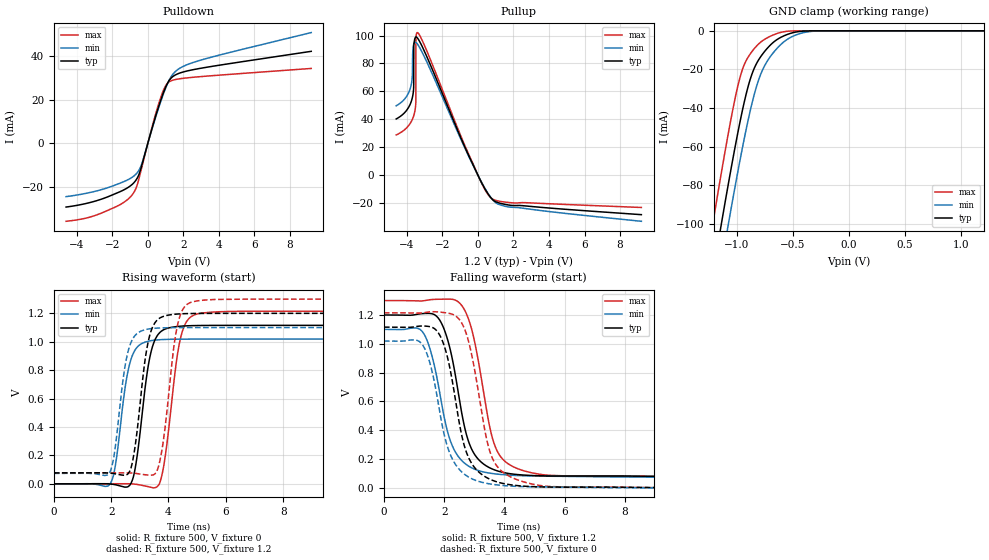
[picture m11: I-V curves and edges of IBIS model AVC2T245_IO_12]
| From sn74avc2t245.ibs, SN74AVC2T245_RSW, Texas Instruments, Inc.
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[Model]   AVC2T245_IO_12
Model_type  I/O
Vinl=0.385
Vinh=0.845
Enable   Active-Low
Vref =   0
Rref =   2000
Cref =   15p
Vmeas =   0.6
| variable   typ   min   max
C_comp   5.09pF   4.44pF   5.69pF
| C_pullup   5.41pF   3.52pF   7.45pF
| C_pulldown   4.96pF   4.40pF   6.21pF
| C_tri-state   5.09pF   4.44pF   5.69pF
[Temperature Range]   40   100   -40
| Ambient temperature   25   85   -40
[Voltage range]   1.2   1.1   1.3
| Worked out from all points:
|   slope of the pulldown table from 0 to 0.18 V, typ, clamps not added: 34.6 ohm
|   slope of the pullup table from 0 to 0.18 V, typ, clamps not added: 38.5 ohm
|   GND clamp passes 1 mA (typ) near -0.50 V on its own axis
|   rising waveform, R_fixture 500, V_fixture 0: 20-80 % time 426ps typ, 410ps min, 445ps max; typ from 0 V to 1.12 V
|   falling waveform, R_fixture 500, V_fixture 1.2: 20-80 % time 663ps typ, 677ps min, 669ps max; typ from 1.2 V to 0.077 V
|   rising waveform, R_fixture 500, V_fixture 1.2: 20-80 % time 407ps typ, 391ps min, 423ps max; typ from 0.077 V to 1.2 V
|   falling waveform, R_fixture 500, V_fixture 0: 20-80 % time 659ps typ, 674ps min, 671ps max; typ from 1.12 V to 0 V
[GND Clamp]
| AVC2T245_IO_12
|   Voltage   I(typ)   I(min)   I(max)
-4.6V     -1.415A    -1.424A    -1.406A
-1.23V    -132.8mA   -153.7mA   -106.4mA
-1.205V   -124mA     -145mA     -97.63mA
-1.135V   -99.98mA   -121mA     -73.45mA
-1.08V    -81.59mA   -102.5mA   -55.25mA
-1.065V   -76.69mA   -97.53mA   -50.48mA
-960mV    -44.57mA   -64.28mA   -22.28mA
-855mV    -21.19mA   -35.79mA   -10.15mA
-740mV    -9.962mA   -17.01mA   -4.06mA
-565mV    -2.263mA   -5.08mA    -343.5uA
-280mV    -5.263uA   -97.56uA   -11.86nA
1.2V      717.1pA    866.1nA    57.51pA
[Pulldown]
| AVC2T245_IO_12
|   Voltage   I(typ)   I(min)   I(max)
-4.6V     -28.98mA   -24.24mA   -35.47mA
-2.64V    -25.46mA   -21.11mA   -31.83mA
-1.485V   -21.69mA   -17.85mA   -27.52mA
-865mV    -18.55mA   -15.32mA   -23.28mA
-620mV    -16.14mA   -13.56mA   -19.46mA
-375mV    -11.06mA   -10.1mA    -12.1mA
650mV     17.79mA    17.17mA    19mA
955mV     24.67mA    24.15mA    25.54mA
1.215V    28.82mA    29mA       28.13mA
1.685V    31.71mA    33.63mA    29.31mA
2.565V    33.61mA    36.91mA    30.15mA
9.2V      41.96mA    50.5mA     34.16mA
[Pullup]
| AVC2T245_IO_12
|   Voltage   I(typ)   I(min)   I(max)
-4.6V     40.27mA    49.7mA     28.8mA
-3.925V   48.11mA    58.42mA    35.16mA
-3.69V    55.6mA     72.23mA    40.01mA
-3.67V    56.81mA    87.93mA    40.6mA
-3.615V   63.37mA    93.79mA    42.54mA
-3.61V    92.97mA    93.99mA    42.74mA
-3.555V   97.57mA    95.14mA    45.5mA
-3.495V   98.98mA    95.13mA    52.19mA
-3.49V    99mA       95.09mA    98.25mA
-3.4V     98.18mA    93.83mA    102.1mA
760mV     -16.62mA   -16.55mA   -16.53mA
9.2V      -28.27mA   -33.02mA   -23.12mA
[Ramp]
| AVC2T245_IO_12
| variable   typ   min   max
dV/dt_r   0.68/4.41E-10   0.62/4.22E-10   0.75/4.59E-10
dV/dt_f   0.68/6.73E-10   0.62/6.87E-10   0.74/6.81E-10
R_load = 500
[Rising Waveform]
| AVC2T245_IO_12
R_fixture =   500
C_fixture =   0
L_fixture =   0
V_fixture =   0
V_fixture_min = 0
V_fixture_max = 0
|   Time   V(typ)   V(min)   V(max)
0s        17.24nV    2.655uV    192.3pV
1.98ns    -1.134mV   4.283mV    926.4uV
2.67ns    -4.763mV   861.1mV    467.3uV
2.895ns   179.3mV    958.5mV    -3.854mV
3.32ns    859.5mV    1.005V     -20.93mV
3.64ns    1.052V     1.014V     -12.45mV
3.855ns   1.087V     1.016V     150.7mV
4.44ns    1.11V      1.018V     1.041V
5.135ns   1.115V     1.019V     1.201V
38.12ns   1.115V     1.019V     1.215V
[Falling Waveform]
| AVC2T245_IO_12
R_fixture =   500
C_fixture =   0
L_fixture =   0
V_fixture =   1.2
V_fixture_min = 1.1
V_fixture_max = 1.3
|   Time   V(typ)   V(min)   V(max)
0s        1.2V       1.1V       1.3V
1.33ns    1.21V      1.068V     1.299V
1.625ns   1.207V     892.4mV    1.308V
2ns       1.101V     491.9mV    1.31V
2.535ns   580mV      200.6mV    1.278V
2.97ns    246.7mV    133.5mV    1.054V
3.5ns     140.7mV    102.7mV    437.2mV
3.745ns   119.5mV    95.9mV     262.8mV
5.165ns   83.94mV    81.4mV     94.67mV
38.12ns   77.01mV    73.71mV    77.16mV
[Rising Waveform]
| AVC2T245_IO_12
R_fixture =   500
C_fixture =   0
L_fixture =   0
V_fixture =   1.2
V_fixture_min = 1.1
V_fixture_max = 1.3
|   Time   V(typ)   V(min)   V(max)
0s        77.01mV    73.71mV    77.16mV
1.955ns   75.63mV    83.61mV    77.89mV
2.61ns    76.29mV    946.3mV    76.98mV
2.84ns    269.2mV    1.045V     73.94mV
3.25ns    955.8mV    1.088V     62.64mV
3.575ns   1.146V     1.096V     80.26mV
3.825ns   1.179V     1.098V     308.2mV
4.335ns   1.196V     1.099V     1.134V
5.015ns   1.199V     1.1V       1.288V
38.12ns   1.2V       1.1V       1.3V
[Falling Waveform]
| AVC2T245_IO_12
R_fixture =   500
C_fixture =   0
L_fixture =   0
V_fixture =   0
V_fixture_min = 0
V_fixture_max = 0
|   Time   V(typ)   V(min)   V(max)
0s        1.115V     1.019V     1.215V
1.305ns   1.123V     985.6mV    1.215V
1.59ns    1.115V     815.8mV    1.222V
1.975ns   1.002V     394.3mV    1.217V
2.475ns   483.4mV    135mV      1.176V
2.88ns    182mV      67.36mV    957.5mV
3.385ns   74.57mV    32.51mV    364.2mV
3.635ns   50.02mV    23.68mV    191.7mV
5.185ns   6.809mV    6.882mV    16.51mV
38.12ns   89.99nV    2.835uV    85.37nV
